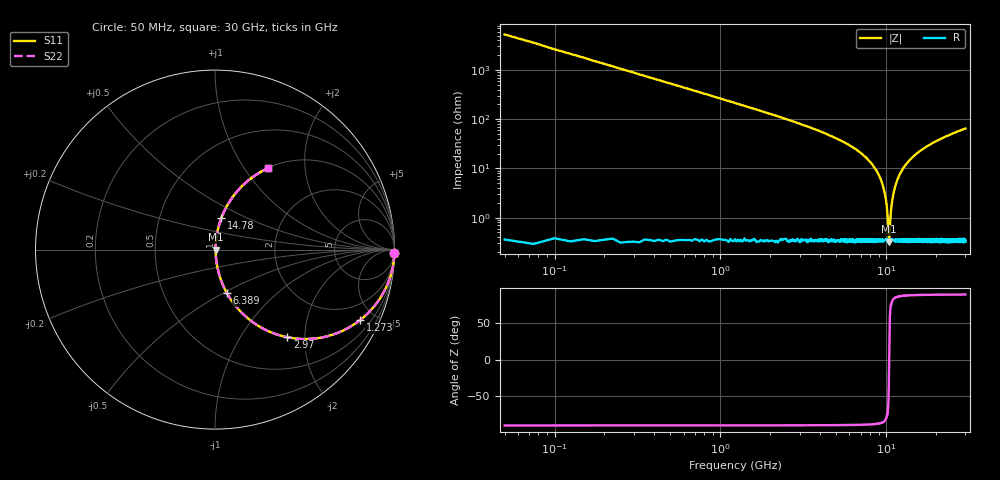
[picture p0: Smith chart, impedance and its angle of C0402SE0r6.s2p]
!	AVX Thin Film Operation 	Date: April 2014
!	Description: Accu-P® Series, Thin Film  SMD RF Capacitor
!	Part Number: 04021J0R6PBSTR
# MHZ S MA R 50
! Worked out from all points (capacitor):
!   1201 points, 50 MHz to 30 GHz, reference 50 ohm
!   read as one part in series: C = 600 fF near 199.8 MHz
!   lowest |Z| = 322 mohm at 10.41 GHz (marker M1)
!   series resonance near 10.4 GHz, so ESL is about 390 pH
!   S11 on the Smith chart (normalised r, x): 50 MHz: open; 1.273 GHz: 1.01, -4.10; 2.97 GHz: 1.01, -1.64; 6.389 GHz: 1.01, -0.52; 14.78 GHz: 1.01, +0.37; 30 GHz: 1.01, +1.29
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50  1 -1.1  0.019 88.9  0.019 88.9  1 -1.1
274.625  0.995 -5.9  0.103 84.1  0.103 84.1  0.995 -5.9
474.292  0.984 -10.2  0.176 79.8  0.176 79.8  0.984 -10.2
823.708  0.954 -17.3  0.298 72.6  0.298 72.6  0.954 -17.3
1272.958  0.898 -26.0  0.438 63.9  0.438 63.9  0.898 -26.0
2970.125  0.633 -50.5  0.772 39.3  0.772 39.3  0.633 -50.5
5041.667  0.372 -67.7  0.925 21.9  0.925 21.9  0.372 -67.7
6389.417  0.25 -74.8  0.965 14.5  0.965 14.5  0.25 -74.8
8885.25  0.08 -83.0  0.993 4.6  0.993 4.6  0.08 -83.0
9609.042  0.041 -82.9  0.996 2.3  0.996 2.3  0.041 -82.9
10058.29  0.018 -77.8  0.996 1.0  0.996 1.0  0.018 -77.8
10307.88  0.005837 -53.9  0.997 0.3  0.997 0.3  0.005837 -53.9
10407.71  0.003423 2.8  0.997 -0.0  0.997 -0.0  0.003423 2.8
10507.54  0.006072 55.4  0.997 -0.3  0.997 -0.3  0.006072 55.4
10906.88  0.024 80.5  0.996 -1.4  0.996 -1.4  0.024 80.5
11555.79  0.053 83.3  0.995 -3.1  0.995 -3.1  0.053 83.3
12828.67  0.107 82.1  0.991 -6.1  0.991 -6.1  0.107 82.1
14775.42  0.179 78.6  0.98 -10.3  0.98 -10.3  0.179 78.6
15025  0.188 78.2  0.979 -10.8  0.979 -10.8  0.188 78.2
20016.67  0.336 69.8  0.939 -19.6  0.939 -19.6  0.336 69.8
25033.29  0.451 62.8  0.889 -26.8  0.889 -26.8  0.451 62.8
30000  0.542 56.9  0.838 -32.8  0.838 -32.8  0.542 56.9
